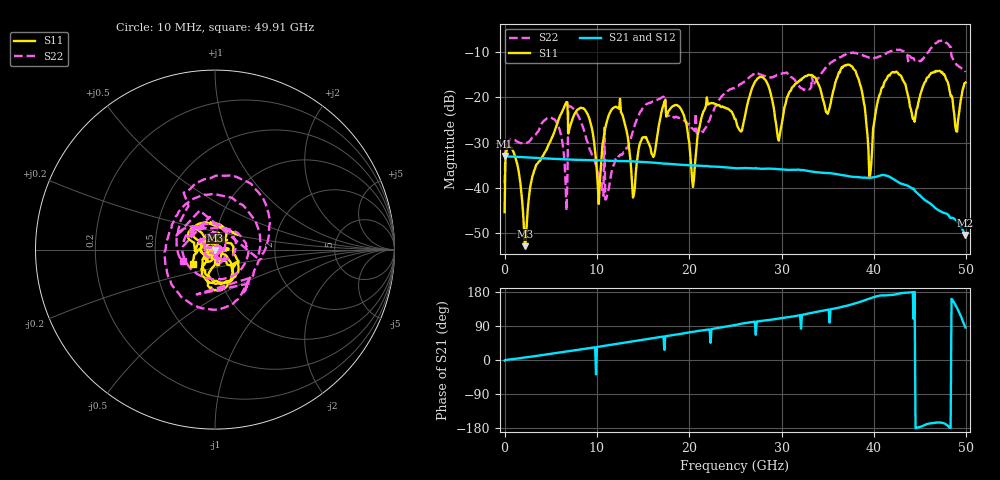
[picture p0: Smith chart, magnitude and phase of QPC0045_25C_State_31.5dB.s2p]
!File name = QPC0045_25C_State_31.5dB.s2p
!Date Time: 2024/05/02 05:42:16 AM
!Cal Ref Plane:TRL
!TEMP = 25C
!Vdd(V) = 3.15
!Vss(V) = 0.000
# GHz  S  DB  R  50
!%	Freq(GHz)  S11(dB)  S11(deg)  S21(dB)  S21(deg)  S12(dB)  S12(deg)  S22(dB)  S22(deg)
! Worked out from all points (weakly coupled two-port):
!   500 points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, 10 MHz to 49.91 GHz, reference 50 ohm
!   highest |S21| = -32.97 dB at 10 MHz (marker M1); lowest = -50.4 dB at 49.91 GHz (marker M2)
!   lowest |S11| = -52.9 dB at 2.21 GHz (marker M3), VSWR 1.00, Z = 50.2 - j0.156 ohm
!   |S11| at or under -10 dB: start of sweep to end of sweep
!   |S22| runs from -45.1 to -7.5 dB; largest |S21 - S12| = 7e-05
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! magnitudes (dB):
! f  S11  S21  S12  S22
! 10 MHz  -45.4  -33.0  -33.0  -39.0
! 910 MHz  -31.8  -33.1  -33.1  -29.2
! 2.21 GHz  -52.9  -33.3  -33.3  -30.1
! 5.31 GHz  -28.1  -33.6  -33.6  -24.8
! 6.61 GHz  -21.5  -33.7  -33.7  -38.9
! 7.11 GHz  -26.3  -33.8  -33.8  -22.0
! 8.41 GHz  -22.4  -33.9  -33.9  -26.1
! 10.21 GHz  -43.5  -33.9  -33.9  -37.1
! 11.11 GHz  -25.2  -34.0  -34.0  -41.6
! 12.71 GHz  -23.7  -34.1  -34.1  -32.7
! 14.01 GHz  -41.4  -34.2  -34.2  -26.7
! 16.71 GHz  -26.3  -34.5  -34.5  -20.4
! 19.01 GHz  -22.3  -34.9  -34.9  -24.7
! 20.41 GHz  -39.8  -35.0  -35.0  -27.0
! 21.91 GHz  -20.0  -35.2  -35.2  -26.3
! 25.01 GHz  -24.8  -35.7  -35.7  -17.9
! 33.31 GHz  -15.1  -36.4  -36.4  -15.3
! 37.81 GHz  -13.8  -37.6  -37.6  -10.2
! 39.61 GHz  -37.0  -37.8  -37.8  -11.3
! 41.61 GHz  -15.1  -37.5  -37.5  -10.1
! 48.91 GHz  -27.4  -47.2  -47.1  -12.7
! 49.91 GHz  -16.8  -50.4  -50.4  -14.4
